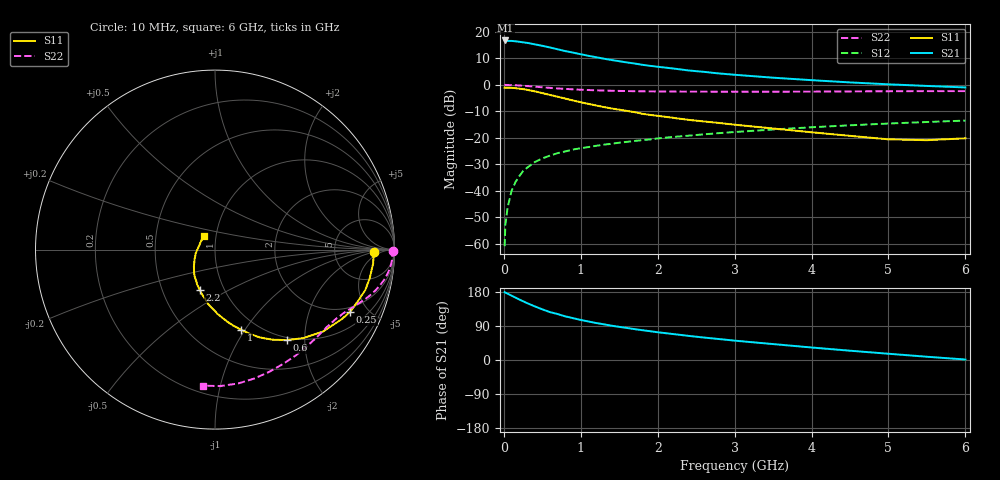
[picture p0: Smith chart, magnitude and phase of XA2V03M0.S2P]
! SIEMENS Discrete & RF Semiconductors
! BFY180
! Si NPN RF Bipolar Junction Transistor in MICRO-X
! VCE = 2 V  IC = 3 mA
! Common Emitter S-Parameters:  May  1997
# GHz  S  MA  R  50
!  f  S11  S21  S12  S22
! GHz  MAG  ANG  MAG  ANG  MAG  ANG  MAG  ANG
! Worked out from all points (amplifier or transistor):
!   36 points, 10 MHz to 6 GHz, reference 50 ohm
!   highest |S21| = 16.8 dB at 20 MHz (marker M1)
!   |S21| within 3 dB of that: start of sweep to 650.9 MHz
!   unconditionally stable (mu >= 1): 1.642 GHz to end of sweep
!   at 250 MHz: K = 0.22, MSG = 24.3 dB, |S12| = -32.6 dB
!   at 1.4 GHz: K = 0.93, MSG = 15.8 dB, |S12| = -22.3 dB
!   at 6 GHz: K = 1.13, MAG = 4.1 dB, |S12| = -13.5 dB
!   S11 on the Smith chart (normalised r, x): 10 MHz: 16, -2; 250 MHz: 1.73, -3.83; 600 MHz: 0.95, -1.65; 1 GHz: 0.84, -0.96; 2.2 GHz: 0.77, -0.36; 6 GHz: 0.87, +0.13
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0.01  0.8857 -0.9  6.775 179.0  0.0009 90.2  0.9891 -0.3
0.02  0.8838 -2.0  6.883 177.7  0.0023 88.9  0.9971 -0.7
0.05  0.8846 -5.0  6.737 175.0  0.0049 85.7  0.9895 -2.0
0.1  0.8766 -10.4  6.747 169.8  0.0099 85.3  0.9868 -4.0
0.15  0.867 -15.1  6.639 164.8  0.0145 81.4  0.9806 -5.9
0.25  0.8293 -24.7  6.343 155.0  0.0235 75.7  0.9612 -9.6
0.3  0.8054 -28.8  6.208 150.3  0.0271 73.4  0.9488 -11.2
0.4  0.7551 -37.2  5.826 141.7  0.0347 68.8  0.9251 -14.0
0.5  0.6977 -44.9  5.457 133.6  0.0408 64.9  0.8992 -16.6
0.6  0.6443 -51.5  5.071 126.4  0.0462 62.1  0.8763 -18.7
0.8  0.5499 -62.9  4.33 115.1  0.0554 58.0  0.8381 -22.2
1  0.4692 -72.0  3.78 105.7  0.0637 54.4  0.8084 -25.2
1.1  0.437 -76.3  3.528 101.7  0.0669 53.5  0.7972 -26.5
1.3  0.3803 -84.1  3.116 94.2  0.0742 51.9  0.7793 -29.3
1.5  0.3398 -90.4  2.792 87.4  0.0809 50.4  0.7676 -32.0
1.8  0.284 -100.6  2.389 78.7  0.0905 49.3  0.7554 -36.0
2.2  0.2385 -111.2  2.037 68.5  0.1038 46.4  0.7475 -41.6
2.8  0.1904 -126.0  1.639 55.3  0.1226 42.9  0.7424 -49.7
3.5  0.1499 -141.6  1.364 42.0  0.1433 38.2  0.7415 -59.2
4.5  0.1089 -169.8  1.111 24.5  0.1722 30.7  0.7509 -73.0
5.5  0.0902 154.6  0.953 8.6  0.1988 22.8  0.7608 -87.7
6  0.0978 130.3  0.893 1.3  0.2114 18.6  0.7613 -95.0
